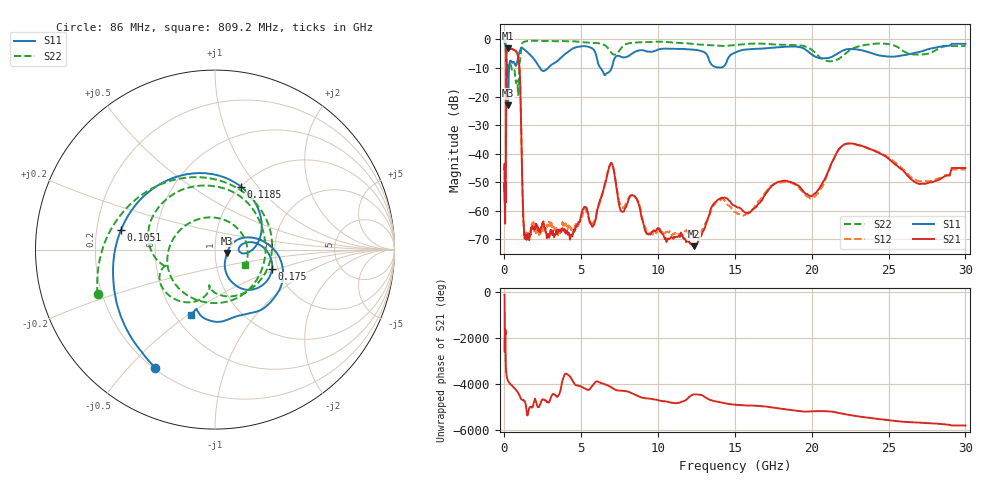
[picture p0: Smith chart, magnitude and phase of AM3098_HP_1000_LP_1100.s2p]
! Date/Time: Thu, Feb 28, 2019 8:40 AM
! Network Analyzer: Agilent Technologies E8364B Rev: A.07.50.67
! Sweep from 0.010 to 30.000 GHz, 1601 Points, Sweep Type: LOG
! Power Supply: 5.022 V, 0.002 A
# Hz S DB R 50
!freq MagS11 AngS11 MagS21 AngS21 MagS12 AngS12 MagS22 AngS22
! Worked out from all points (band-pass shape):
!   1601 points, 10 MHz to 30 GHz, reference 50 ohm
!   highest |S21| = -3.05 dB at 242.3 MHz (marker M1); lowest = -72.4 dB at 12.31 GHz (marker M2)
!   |S21| within 3 dB of the highest: 128 MHz to 885.1 MHz (757.1 MHz wide, 149 % of centre)
!   lowest |S11| = -23.1 dB at 239.9 MHz (marker M3), VSWR 1.15, Z = 57.2 - j2.07 ohm
!   |S11| at or under -10 dB: 192 MHz to 300.1 MHz (108.1 MHz wide, 43.9 % of centre); 2.321 GHz to 2.837 GHz (515.4 MHz wide, 20 % of centre); 6.252 GHz to 6.975 GHz (722.9 MHz wide, 10.9 % of centre)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
!   |S22| runs from -19.5 to -0.5 dB; largest |S21 - S12| = 0.011
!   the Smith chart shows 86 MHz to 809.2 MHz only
!   S11 on the Smith chart (normalised r, x): 86 MHz: 0.21, -0.59; 105.1 MHz: 0.31, +0.09; 118.5 MHz: 1.00, +0.82; 175 MHz: 1.86, -0.45; 809.2 MHz: 0.60, -0.51
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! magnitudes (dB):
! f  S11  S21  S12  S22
! 10 MHz  -0.4  -45.6  -45.8  -0.6
! 38.04 MHz  -0.5  -58.7  -60.4  -1.0
! 86 MHz  -2.6  -52.9  -54.4  -3.1
! 105.1 MHz  -5.4  -27.3  -27.0  -7.0
! 118.5 MHz  -8.4  -10.7  -10.7  -10.1
! 144.7 MHz  -16.8  -4.2  -4.2  -13.0
! 175 MHz  -9.5  -3.7  -3.7  -8.9
! 239.9 MHz  -23.1  -3.0  -3.0  -11.0
! 242.3 MHz  -22.9  -3.0  -3.0  -10.9
! 550.5 MHz  -8.0  -3.5  -3.5  -10.7
! 809.2 MHz  -8.3  -4.7  -4.7  -14.5
! 1.009 GHz  -4.1  -13.0  -13.0  -7.6
! 1.289 GHz  -3.6  -68.2  -68.3  -0.8
! 2.084 GHz  -8.1  -65.3  -67.0  -0.5
! 5.725 GHz  -3.2  -65.6  -64.2  -1.2
! 6.89 GHz  -10.9  -43.7  -43.5  -4.2
! 7.926 GHz  -6.2  -58.5  -57.1  -1.6
! 12.31 GHz  -3.6  -72.4  -68.1  -1.6
! 14.02 GHz  -9.9  -55.9  -56.4  -2.2
! 20.1 GHz  -5.6  -54.3  -55.4  -4.1
! 22.56 GHz  -3.4  -36.4  -36.4  -3.5
! 30 GHz  -1.6  -45.0  -45.5  -2.3
